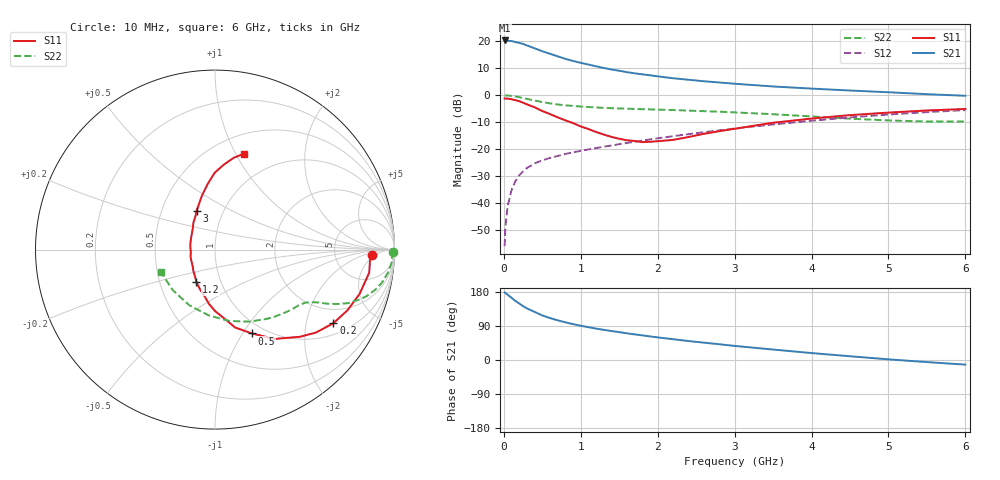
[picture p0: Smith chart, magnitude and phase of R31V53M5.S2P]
! SIEMENS Small Signal Semiconductors
! BFR181
! Si NPN RF Bipolar Junction Transistor in SOT23
! VCE = 1.5 V  IC = 3.5 mA
! Common Emitter S-Parameters:  May  1996
# GHz  S  MA  R  50
!  f  S11  S21  S12  S22
! GHz  MAG  ANG  MAG  ANG  MAG  ANG  MAG  ANG
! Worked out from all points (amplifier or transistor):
!   36 points, 10 MHz to 6 GHz, reference 50 ohm
!   highest |S21| = 20.3 dB at 10 MHz (marker M1)
!   |S21| within 3 dB of that: start of sweep to 408.4 MHz
!   unconditionally stable (mu >= 1): 1.23 GHz to 3.159 GHz
!   at 250 MHz: K = 0.35, MSG = 23.6 dB, |S12| = -28.2 dB
!   at 1.4 GHz: K = 1.04, MAG = 12.8 dB, |S12| = -18.6 dB
!   at 6 GHz: K = 0.87, MSG = 2.7 dB, |S12| = -5.5 dB
!   S11 on the Smith chart (normalised r, x): 10 MHz: 14, -3; 200 MHz: 1.40, -2.89; 500 MHz: 0.87, -1.10; 1.2 GHz: 0.77, -0.29; 3 GHz: 0.75, +0.34; 6 GHz: 0.70, +1.08
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0.01  0.8729 -1.8  10.36 178.5  0.0016 98.8  0.993 -0.7
0.02  0.8657 -3.2  10.2 176.6  0.0036 92.2  0.9873 -1.6
0.05  0.8688 -8.5  10.22 172.0  0.0089 84.7  0.9885 -3.9
0.1  0.8428 -17.0  10.11 164.2  0.0174 80.9  0.9724 -7.6
0.15  0.8124 -24.5  9.691 155.9  0.0257 76.2  0.9487 -11.2
0.2  0.7766 -31.9  9.346 149.1  0.0328 72.9  0.9202 -14.1
0.25  0.7281 -39.4  8.933 142.1  0.0389 69.0  0.8882 -16.7
0.3  0.6786 -45.7  8.383 136.2  0.0449 67.2  0.8555 -18.9
0.4  0.5989 -56.2  7.414 126.9  0.0547 63.2  0.7997 -21.9
0.5  0.5102 -66.3  6.542 117.6  0.0623 61.1  0.7482 -23.9
0.6  0.4482 -75.5  5.872 110.6  0.069 59.5  0.7073 -25.3
0.8  0.3435 -89.7  4.731 99.4  0.0816 58.3  0.6517 -26.9
0.9  0.3049 -96.3  4.316 94.7  0.0877 58.6  0.634 -27.6
1.1  0.2364 -110.8  3.703 86.6  0.0992 59.0  0.6048 -29.0
1.2  0.2086 -119.7  3.439 82.7  0.1051 59.5  0.594 -29.7
1.6  0.1466 -153.0  2.68 70.4  0.1307 60.2  0.5641 -33.0
2.2  0.1489 153.2  2.066 54.9  0.1745 59.7  0.5325 -40.2
3  0.2396 115.3  1.636 37.2  0.2414 56.3  0.4819 -53.1
3.5  0.3095 103.6  1.455 27.6  0.2875 52.6  0.4456 -64.3
4.5  0.4285 90.2  1.225 9.9  0.3886 42.7  0.3682 -95.5
5.5  0.5226 78.4  1.047 -5.5  0.4868 29.9  0.3261 -136.1
6  0.5575 73.3  0.979 -12.2  0.5308 22.6  0.3274 -157.8
